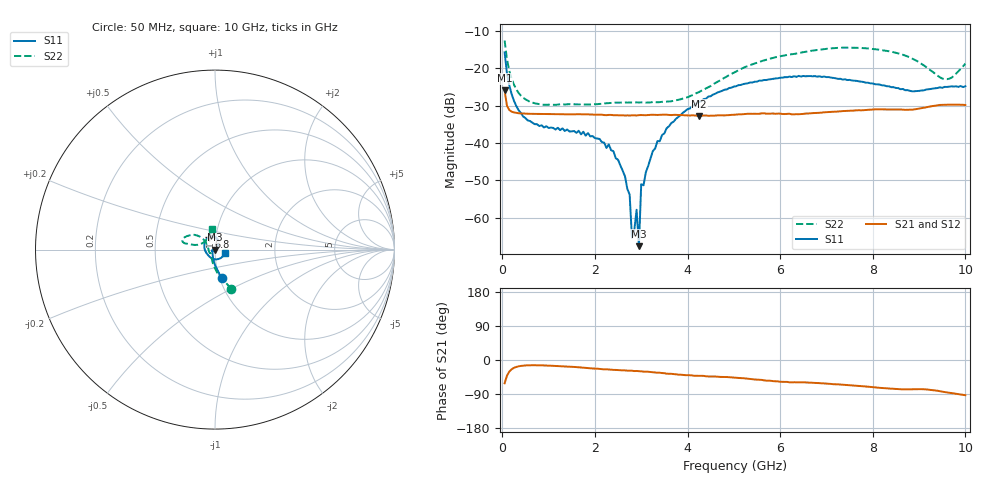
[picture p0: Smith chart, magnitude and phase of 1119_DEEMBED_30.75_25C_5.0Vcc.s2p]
!Hittite Microwave Corp.
!Digital Attenuator/PhaseShifter Rev 1.4.0
!Filename: C:\DATA\DATA\1119_DEEMBED_30.75_25C_5.0Vcc.s2p
!VNA ID: Agilent Technologies,N5224A,MY51441122,A.10.45.03
!Device type:
!2 Port Calibration.
!Temp(C): 25
!Lot Number:
!Serial Number:
!Operator:
!Misc:
!Attenuator:  30.750
# GHZ S DB R 50.0
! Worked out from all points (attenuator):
!   200 points, 50 MHz to 10 GHz, reference 50 ohm
!   highest |S21| = -25.89 dB at 50 MHz (marker M1); lowest = -32.7 dB at 4.25 GHz (marker M2)
!   lowest |S11| = -67.6 dB at 2.95 GHz (marker M3), VSWR 1.00, Z = 50 + j0.00581 ohm
!   |S11| at or under -10 dB: start of sweep to end of sweep
!   |S22| runs from -29.8 to -12.6 dB; largest |S21 - S12| = 0.00012
!   S11 on the Smith chart (normalised r, x): 50 MHz: 1.02, -0.33; 6.8 GHz: 0.92, +0.13; 10 GHz: 1.11, -0.04
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0.05  -15.75 -77.1  -25.89 -61.4  -25.89 -61.4  -12.56 -67.6
0.1  -21.25 -90.1  -30.01 -41.7  -29.99 -41.7  -17.51 -84.0
0.2  -26.85 -104.3  -31.60 -24.6  -31.59 -24.6  -22.78 -100.6
0.45  -32.90 -127.4  -32.10 -14.9  -32.11 -14.9  -27.87 -121.4
1.75  -36.98 -164.2  -32.34 -20.4  -32.32 -20.3  -29.67 -140.9
2.3  -40.39 -170.5  -32.48 -25.0  -32.48 -25.0  -29.31 -149.4
2.5  -44.49 -168.4  -32.60 -26.6  -32.60 -26.6  -29.21 -151.7
2.75  -53.83 -173.8  -32.65 -27.9  -32.66 -28.1  -29.15 -155.6
2.8  -65.34 -125.3  -32.58 -28.4  -32.59 -28.4  -29.15 -156.7
2.85  -63.42 -171.1  -32.60 -29.2  -32.61 -29.2  -29.17 -158.0
2.9  -57.86 21.9  -32.63 -28.9  -32.64 -29.0  -29.12 -159.2
2.95  -67.60 8.0  -32.54 -29.4  -32.54 -29.5  -29.15 -160.3
3  -51.01 32.5  -32.52 -30.0  -32.53 -30.1  -29.12 -161.8
3.4  -39.53 51.5  -32.45 -33.6  -32.47 -33.7  -29.06 -173.9
3.65  -34.66 52.4  -32.53 -36.4  -32.54 -36.5  -28.83 177.0
4.25  -28.98 57.4  -32.74 -41.9  -32.76 -42.0  -26.37 152.0
5.05  -24.81 73.3  -32.40 -46.7  -32.42 -46.7  -20.83 138.5
6.7  -22.15 115.1  -32.00 -60.2  -32.01 -60.2  -15.27 153.8
6.8  -22.24 117.8  -31.95 -61.0  -31.97 -61.0  -15.12 155.1
8.35  -24.82 178.6  -31.02 -75.2  -31.02 -75.2  -15.45 168.1
9.55  -24.98 -69.8  -29.76 -84.6  -29.77 -84.6  -22.92 138.1
10  -24.82 -19.8  -29.83 -92.9  -29.84 -92.9  -18.76 98.2
